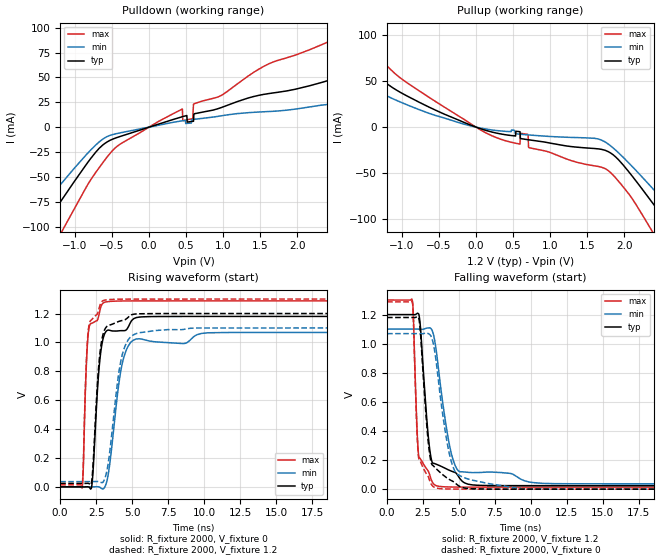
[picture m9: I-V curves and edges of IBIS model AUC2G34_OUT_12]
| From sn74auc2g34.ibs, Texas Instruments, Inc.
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[Model]   AUC2G34_OUT_12
Model_type  Output
Vref =   0
Rref =   2000
Cref =   15p
Vmeas =   0.6
| variable   typ   min   max
C_comp   5.96pF   2.40pF   15.73pF
| C_pullup   5.54pF   2.40pF   15.73pF
| C_pulldown   6.39pF   4.23pF   14.99pF
[Temperature Range]   40   100   -40
| Ambient temperature   25   85   -40
[Voltage range]   1.2   1.1   1.3
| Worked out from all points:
|   slope of the pulldown table from 0 to 0.18 V, typ, clamps not added: 42.2 ohm
|   slope of the pullup table from 0 to 0.18 V, typ, clamps not added: 38.7 ohm
|   rising waveform, R_fixture 2000, V_fixture 0: 20-80 % time 477ps typ, 805ps min, 284ps max; typ from 0 V to 1.18 V
|   falling waveform, R_fixture 2000, V_fixture 1.2: 20-80 % time 564ps typ, 955ps min, 285ps max; typ from 1.2 V to 0.024 V
|   rising waveform, R_fixture 2000, V_fixture 1.2: 20-80 % time 468ps typ, 799ps min, 278ps max; typ from 0.024 V to 1.2 V
|   falling waveform, R_fixture 2000, V_fixture 0: 20-80 % time 562ps typ, 962ps min, 283ps max; typ from 1.18 V to 0 V
[Pulldown]
| AUC2G34_OUT_12
|   Voltage   I(typ)   I(min)   I(max)
-3.6V     -338.8mA   -281.7mA   -417.7mA
-1.81V    -142.6mA   -113.7mA   -188.4mA
-1.485V   -106.8mA   -83.81mA   -145.9mA
-1.225V   -78.22mA   -60.33mA   -111.4mA
-675mV    -21.44mA   -15mA      -40.91mA
-395mV    -9.496mA   -5.836mA   -17.3mA
450mV     10.5mA     6.398mA    18.24mA
590mV     5.848mA    7.731mA    8.546mA
605mV     12.96mA    7.861mA    23.36mA
2.86V     55.95mA    19.1mA     100.7mA
3.425V    44.58mA    20.08mA    119.3mA
7.2V      57.06mA    26.83mA    108mA
[Pullup]
| AUC2G34_OUT_12
|   Voltage   I(typ)   I(min)   I(max)
-3.6V     223.7mA    100.2mA    290.4mA
-2.7V     158.2mA    65.85mA    204.5mA
-2.11V    110mA      77.74mA    148.3mA
-1.675V   77.42mA    55.44mA    108mA
-1.025V   38.18mA    27.56mA    53.96mA
50mV      -1.427mA   -842.9uA   -2.489mA
700mV     -13.68mA   -8.451mA   -7.891mA
1.78V     -26.51mA   -18.11mA   -47.11mA
2.4V      -84.42mA   -68.22mA   -116.5mA
2.695V    -116.8mA   -94.89mA   -156.2mA
3.045V    -155.7mA   -127.2mA   -203mA
7.2V      -616.4mA   -522.4mA   -745.9mA
[Ramp]
| AUC2G34_OUT_12
| variable   typ   min   max
dV/dt_r   0.72/4.82E-10   0.65/8.15E-10   0.78/2.87E-10
dV/dt_f   0.71/5.70E-10   0.64/9.60E-10   0.78/2.89E-10
R_load = 2000
[Rising Waveform]
| AUC2G34_OUT_12
R_fixture =   2000
C_fixture =   0
L_fixture =   0
V_fixture =   0
V_fixture_min = 0
V_fixture_max = 0
|   Time   V(typ)   V(min)   V(max)
0s        6.566nV    27.84nV    704.7pV
1.53ns    -5.416uV   -1.013uV   -7.893mV
1.875ns   792.5uV    -11.57uV   953mV
2.175ns   -6.094mV   22.52uV    1.131V
2.68ns    793.8mV    -49.91uV   1.183V
3.025ns   1.041V     -11.57mV   1.275V
3.395ns   1.085V     122mV      1.283V
4.275ns   1.081V     835.5mV    1.287V
5.115ns   1.165V     1.017V     1.287V
23.3ns    1.18V      1.069V     1.287V
[Falling Waveform]
| AUC2G34_OUT_12
R_fixture =   2000
C_fixture =   0
L_fixture =   0
V_fixture =   1.2
V_fixture_min = 1.1
V_fixture_max = 1.3
|   Time   V(typ)   V(min)   V(max)
0s        1.2V       1.1V       1.3V
1.78ns    1.2V       1.1V       1.288V
2.075ns   1.206V     1.1V       445.5mV
2.21ns    1.203V     1.1V       225.6mV
2.92ns    315.5mV    1.109V     112.7mV
3.115ns   192.7mV    1.096V     56.43mV
3.37ns    173.4mV    989.7mV    26.52mV
4.305ns   131.3mV    323.5mV    15.18mV
5.025ns   79.2mV     121.6mV    14.26mV
23.3ns    24.01mV    36.66mV    13.87mV
[Rising Waveform]
| AUC2G34_OUT_12
R_fixture =   2000
C_fixture =   0
L_fixture =   0
V_fixture =   1.2
V_fixture_min = 1.1
V_fixture_max = 1.3
|   Time   V(typ)   V(min)   V(max)
0s        23.98mV    36.64mV    13.86mV
1.53ns    23.97mV    36.64mV    7.51mV
1.87ns    24.68mV    36.63mV    971.1mV
2.165ns   25.05mV    36.66mV    1.155V
2.65ns    801.3mV    36.78mV    1.217V
2.99ns    1.06V      34.23mV    1.289V
3.335ns   1.117V     161.3mV    1.296V
4.23ns    1.15V      878.2mV    1.299V
5.12ns    1.195V     1.054V     1.3V
23.3ns    1.2V       1.1V       1.3V
[Falling Waveform]
| AUC2G34_OUT_12
R_fixture =   2000
C_fixture =   0
L_fixture =   0
V_fixture =   0
V_fixture_min = 0
V_fixture_max = 0
|   Time   V(typ)   V(min)   V(max)
0s        1.18V      1.069V     1.287V
1.77ns    1.18V      1.069V     1.277V
1.83ns    1.18V      1.069V     1.179V
2.075ns   1.185V     1.069V     417.8mV
2.21ns    1.175V     1.069V     211mV
2.88ns    313mV      1.069V     83.77mV
3.29ns    153.3mV    964mV      12.94mV
4.325ns   67.24mV    248.6mV    1.11mV
5.235ns   11.24mV    84.57mV    273.9uV
23.3ns    31.41uV    9.502uV    12.2uV
